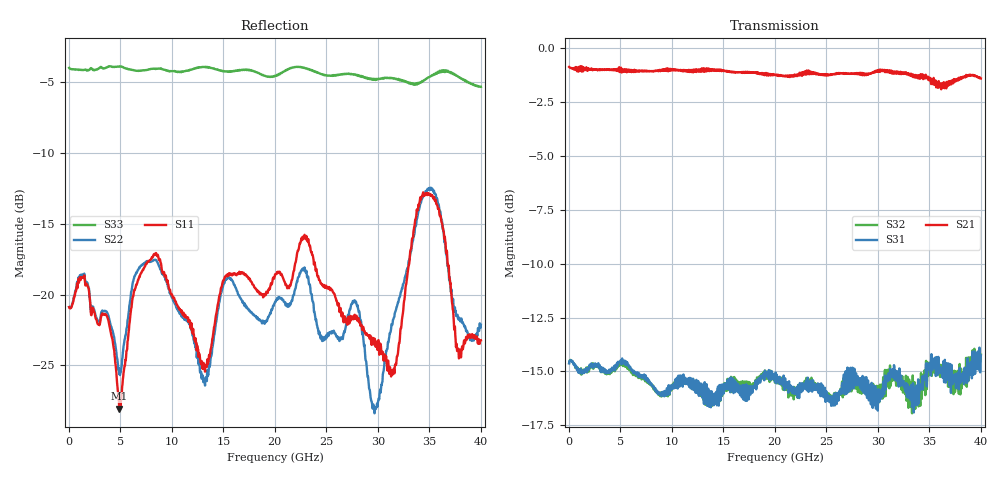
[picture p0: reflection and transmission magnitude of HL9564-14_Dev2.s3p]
! 1/20/2021 10:08:00 AM
! H:\PRODUCTION_DATA\TEMP_S3P.S3P
! CHANNEL.1
! TR.MEASUREMENT
! CORRECTED.DATA
# GHZ S RI R 50.0
! FREQ.GHZ  S11RE  S11IM  S12RE  S12IM  S13RE  S13IM
!  S21RE  S21IM  S22RE  S22IM  S23RE  S23IM
!  S31RE  S31IM  S32RE  S32IM  S33RE  S33IM
!; PortSelection: Port_123
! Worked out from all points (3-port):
!   1143 points, 35 MHz to 40.01 GHz, reference 50 ohm
!   strongest paths, dB at 35 MHz, 10.01 GHz, 20.02 GHz, 30.03 GHz, 40.01 GHz:
!     S21: -0.9, -1.0, -1.2, -1.1, -1.4
!     S31: -14.6, -15.7, -15.5, -16.2, -14.2
!     S32: -14.6, -15.7, -15.5, -15.7, -14.2
!   lowest |S11| = -28.0 dB at 4.9 GHz (marker M1), VSWR 1.08, Z = 46.2 + j0.66 ohm
!   |S11| at or under -10 dB: start of sweep to end of sweep
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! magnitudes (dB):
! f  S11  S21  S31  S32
! 35 MHz  -20.9  -0.9  -14.6  -14.6
! 4.9 GHz  -28.0  -0.9  -14.6  -14.7
! 8.295 GHz  -17.1  -1.1  -15.8  -15.7
! 13.16 GHz  -25.1  -1.1  -16.0  -16.0
! 15.33 GHz  -18.7  -1.1  -15.8  -15.9
! 20.02 GHz  -18.6  -1.2  -15.5  -15.5
! 27.86 GHz  -21.7  -1.2  -15.2  -15.4
! 29.79 GHz  -23.7  -1.1  -16.2  -16.2
! 35.14 GHz  -12.9  -1.5  -15.2  -15.1
! 40.01 GHz  -23.2  -1.4  -14.2  -14.2
